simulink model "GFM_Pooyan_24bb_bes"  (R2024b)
settings: Solver=FixedStepAuto  StartTime=0.0  StopTime=1  FixedStep=Ts  RelTol=1e-3
model workspace (MAT data in the model file):
  Po = 0
  b1 = 1000.38104695
  b2 = 1006.47399607
  b3 = 1006.95432939
  b4 = 996.322108769
  b5 = 995.669039411
  b6 = 1012.96535236
  b7 = 1007.5422409
  b8 = 993.960341463
  l1 = 8282.83466164
  l10 = 5511.54621883
  l11 = 8516.9845943
  l12 = 3533.51403234
  l13 = 1255.67117866
  l14 = 1105.23671469
  l15 = 955.492069576
  l16 = 1255.83166019
  l2 = 7767.51754481
  l3 = 6680.69860842
  l4 = 3013.93364227
  l5 = 912.604633733
  l6 = 706.803488619
  l7 = 1117.39027011
  l8 = 1674.30810947
  l9 = 1971.00014576
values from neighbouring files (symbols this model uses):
  alpha_p = 0.0005    [initialcondition_gfm_Pooyan.m]    (also in initialcondition_Pooyan.m = 0.0001)
  alpha_q = 0.0001    [initialcondition_gfm_Pooyan.m]    (also in initialcondition_Pooyan.m)
  Cf = 50e-6    (= 5e-05)    [initialcondition_gfm_Pooyan.m]    (also in initialcondition_Pooyan.m)
  I_instant_limit_peak = I_instant_limit_rms * sqrt(2)    [initialcondition_gfm_Pooyan.m]
  I_overload_limit = 1.2 * I_rated_rms    [initialcondition_gfm_Pooyan.m]
  Kicc = 314.159    [initialcondition_gfm_Pooyan.m]    (also in initialcondition_Pooyan.m)
  Kivc = 400    [initialcondition_gfm_Pooyan.m]    (also in initialcondition_Pooyan.m)
  Kpcc = 31.4159    [initialcondition_gfm_Pooyan.m]    (also in initialcondition_Pooyan.m)
  Kpvc = 0.5    [initialcondition_gfm_Pooyan.m]    (also in initialcondition_Pooyan.m)
  Lf = 10e-3    (= 0.01)    [initialcondition_gfm_Pooyan.m]    (also in initialcondition_Pooyan.m)
  Lg = X_BY_R*Rg/(wn)    [initialcondition_gfm_Pooyan.m]    (also in DER_param.m = (X_BY_R_gfl * Rg) / wn_gfl; initialcondition_Pooyan.m)
  Pn = 20000    [initialcondition_gfm_Pooyan.m]    (also in initialcondition_Pooyan.m)
  Qn = 0    [initialcondition_gfm_Pooyan.m]    (also in initialcondition_Pooyan.m)
  R = (3*Vg^2)/(2*Pn)    (= 8.000067)    [initialcondition_gfm_Pooyan.m]    (also in MC2.m = (8760*SS-sum(Tdown))/(8760*SS); initialcondition_Pooyan.m)
  R_extra = (3*Vg^2)/(2*P_extra)    (= 10.666756)    [initialcondition_gfm_Pooyan.m]
  Rf = 0.1    [initialcondition_gfm_Pooyan.m]    (also in initialcondition_Pooyan.m)
  Rg = (3*Vg^2)/(2*SCR*sqrt(1+X_BY_R^2)*Pn)    [initialcondition_gfm_Pooyan.m]    (also in DER_param.m = (3 * Vg_gfl^2) / (2 * SCR_gfl * sqrt(1 + X_BY_R_gfl^2) * Pn_; initialcondition_Pooyan.m)
  tau_p = 0.031415    [initialcondition_gfm_Pooyan.m]    (also in initialcondition_Pooyan.m)
  tau_q = 0.031415    [initialcondition_gfm_Pooyan.m]    (also in initialcondition_Pooyan.m)
  Ts = 50e-6    (= 5e-05)    [initialcondition_gfm_Pooyan.m]    (also in initialcondition_Pooyan.m)
  Vdc = 700    [initialcondition_gfm_Pooyan.m]    (also in initialcondition_Pooyan.m)
  Vg = 326.6    [initialcondition_gfm_Pooyan.m]    (also in initialcondition_Pooyan.m)
  wn = 2*pi*50    (= 314.159265359)    [initialcondition_gfm_Pooyan.m]    (also in initialcondition_Pooyan.m)
undefined symbols (not defined in the file or in its folder): Ion, Lithium
libraries: simulink x6, slpidlib x5, spsThreePhaseBreakerLib x3, spsabctodq0Lib x3, spsGroundLib x3, spsThreePhaseSeriesRLCBranchLib x3, spsThreePhaseVIMeasurementLib x3, spsIGBTDiodeLib x2, spsSeriesRLCBranchLib x2, spsThreePhaseParallelRLCBranchLib x2, spsThreePhaseSourceLib x1, spsBatteryLib x1
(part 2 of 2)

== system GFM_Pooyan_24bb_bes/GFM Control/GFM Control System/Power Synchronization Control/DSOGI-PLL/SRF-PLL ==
  al-be-0 : Inport
  1/2/pi : Gain  Gain=1/(2*pi)
  2 : Constant  Value=2*pi
  3 : Constant  Value=0
  Al_Be_0 to dq0 : Subsystem
  Integrator : Integrator
  Math Function : Math  Operator=mod  SignedPower=on
  "PI " : slpidlib/PID Controller  Controller=PI  Form=Parallel  TimeDomain=Continuous-time  UseExternalTs=off  SampleTime=100e-6  IntegratorMethod=Forward Euler  FilterMethod=Forward Euler  ControllerParametersSource=internal  P=10  I=30  UseKiTs=off  D=0  UseExternalDerivativeSource=off  N=100  UseFilter=on  TunerSelectOption=Transfer Function Based (PID Tuner App)  InitialConditionSource=internal  InitialConditionForIntegrator=0  InitialConditionForFilter=0  DifferentiatorICPrevScaledInput=0  ExternalReset=none  TrackingMode=off  Kt=1  LimitOutput=off  SatLimitsSource=internal  UpperSaturationLimit=inf  LowerSaturationLimit=-inf  LinearizeAsGain=on  AntiWindupMode=none  Kb=1  LimitIntegrator=off  UpperIntegratorSaturationLimit=inf  LowerIntegratorSaturationLimit=-inf  POutMin=[]  POutMax=[]  IOutMin=[]  IOutMax=[]  DOutMin=[]  DOutMax=[]  NOutMin=[]  NOutMax=[]  SumOutMin=[]  SumOutMax=[]  SaturationOutMin=[]  SaturationOutMax=[]  PParamMin=[]  PParamMax=[]  IParamMin=[]  IParamMax=[]  DParamMin=[]  DParamMax=[]  NParamMin=[]  NParamMax=[]  KbParamMin=[]  KbParamMax=[]  KtParamMin=[]  KtParamMax=[]  KbOutMin=[]  KbOutMax=[]  KtOutMin=[]  KtOutMax=[]  IntegratorOutMin=[]  IntegratorOutMax=[]  FilterOutMin=[]  FilterOutMax=[]  SumI1OutMin=[]  SumI1OutMax=[]  SumI2OutMin=[]  SumI2OutMax=[]  SumI3OutMin=[]  SumI3OutMax=[]  SumI4OutMin=[]  SumI4OutMax=[]  SumDOutMin=[]  SumDOutMax=[]  DifferentiatorOutMin=[]  DifferentiatorOutMax=[]  FilterDiffOutCoefMin=[]  FilterDiffOutCoefMax=[]  ReciprocalOutMin=[]  ReciprocalOutMax=[]  SumDenOutMin=[]  SumDenOutMax=[]  SumNumOutMin=[]  SumNumOutMax=[]  DivideOutMin=[]  DivideOutMax=[]  UdiffTsProdOutMin=[]  UdiffTsProdOutMax=[]  NTsProdOutMin=[]  NTsProdOutMax=[]  UintegralTsProdOutMin=[]  UintegralTsProdOutMax=[]  UngainTsProdOutMin=[]  UngainTsProdOutMax=[]  ClampingZeroOutDataTypeStr=Inherit: Inherit via back propagation  ClampingZeroOutMin=[]  ClampingZeroOutMax=[]  FilterDenConstantOutDataTypeStr=Inherit: Inherit via back propagation  FilterDenConstantOutMin=[]  FilterDenConstantOutMax=[]  PCopyOutDataTypeStr=Inherit: Inherit via back propagation  PCopyOutMin=[]  PCopyOutMax=[]  NCopyOutDataTypeStr=Inherit: Inherit via back propagation  NCopyOutMin=[]  NCopyOutMax=[]  IntegratorContinuousStateAttributes=''  IntegratorStateMustResolveToSignalObject=off  IntegratorRTWStateStorageClass=Auto  FilterContinuousStateAttributes=''  FilterStateMustResolveToSignalObject=off  FilterRTWStateStorageClass=Auto  ParallelPVariant=InternalParameters  IdealPVariant=Disabled  IVariant=InternalParameters  DVariant=Disabled  IntegratorVariant=Continuous  SatVariant=Disabled  AWVariant=Passthrough  PCopyVariant=Disabled  TRVariant=Disabled  FdbkBlocksVariant=Forward  IdealPFdbkVariant=Disabled  SatFdbkVariant=Disabled  DerivativeFilterVariant=Disabled  NVariant=Disabled  NCopyVariant=Disabled_SignalSpec  FilterICVariant=Disabled  IntegratorICVariant=InternalICs  ExternalResetVariant=Disabled  TRSumVariant=Passthrough  SumFdbkVariant=Disabled  SumVariant=Sum_PI  TsampFilterVariant=InternalTs  TsampNgainVariant=Passthrough  TsampIntegralVariant=Disabled_SignalSpec  ExternalSaturationOutDataTypeStr=Inherit: Same as second input  DerivativeSourceVariant=Disabled  PreIntVariant=InternalPreInt
  Second-Order Filter : spsSecondOrderFilterLib/Second-Order Filter  FilterType=Lowpass  Fo=5  Zeta=0.707  Ts=0  Initialize=off  Vac_Init="[0,  0,  50]"  Vdc_Init=0  PlotResponse=off  FreqRange=[0, 500, 1]
  Selector : Selector  InputPortWidth=3  IndexOptions=Index vector (dialog)  Indices=1  OutputSizes=1
  Sum1 : Sum  Inputs=|++
  Sum2 : Sum  Inputs=|+-
  w : Constant  Value=100*pi
  theta_pcc : Outport  VectorParamsAs1DForOutWhenUnconnected=off
  f : Outport  Port=2  VectorParamsAs1DForOutWhenUnconnected=off
  w_pcc : Outport  Port=3  VectorParamsAs1DForOutWhenUnconnected=off
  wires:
  1/2/pi/1 -> Second-Order Filter/1
  Integrator/1 -> Al_Be_0 to dq0/2(wt), theta_pcc/1, Math Function/1
  2/1 -> Math Function/2
  Sum1/1 -> Integrator/1, w_pcc/1, 1/2/pi/1
  w/1 -> Sum1/2
  "PI "/1 -> Sum1/1
  Sum2/1 -> "PI "/1
  al-be-0/1 -> Al_Be_0 to dq0/1(Al_Be_0)
  3/1 -> Sum2/2
  Al_Be_0 to dq0/1(dq0) -> Selector/1
  Selector/1 -> Sum2/1
  Second-Order Filter/1 -> f/1

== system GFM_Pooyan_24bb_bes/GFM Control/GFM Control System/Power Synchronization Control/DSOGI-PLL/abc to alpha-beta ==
  abc : Inport
  Gain1 : Gain  Gain=(2/3)  SaturateOnIntegerOverflow=on
  Gain3 : Gain  Gain="[ 1   -1/2   -1/2; 0   sqrt(3)/2   -sqrt(3)/2 ]"  Multiplication=Matrix(K*u) (u vector)  SaturateOnIntegerOverflow=on
  al_be : Outport  VectorParamsAs1DForOutWhenUnconnected=off
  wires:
  abc/1 -> Gain3/1
  Gain1/1 -> al_be/1
  Gain3/1 -> Gain1/1

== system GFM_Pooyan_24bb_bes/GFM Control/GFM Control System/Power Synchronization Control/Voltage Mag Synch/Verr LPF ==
  In : Inport
  Add : Sum  Inputs=+-
  Constant1 : Constant  Value=1 / (2*pi*fc)
  Constant2 : Constant
  Constant3 : Constant
  Divide : Product  Inputs=*/
  LPF : Subsystem  mask(Basic IIR LPF filter){}
      mask help: The output is computed as: y[k] = G * y[k-1] + (1-G) * u[k]
  Weighted Sample Time1 : SampleTimeMath
  Weighted Sample Time2 : SampleTimeMath  TsampMathOp=Ts Only
  Out : Outport
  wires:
  Constant3/1 -> Weighted Sample Time2/1
  Divide/1 -> Add/2  "α"
  Weighted Sample Time2/1 -> Divide/1
  Weighted Sample Time1/1 -> Divide/2
  Constant1/1 -> Weighted Sample Time1/1
  Constant2/1 -> Add/1
  In/1 -> LPF/1(In)
  LPF/1(Out) -> Out/1
  Add/1 -> LPF/2(G)

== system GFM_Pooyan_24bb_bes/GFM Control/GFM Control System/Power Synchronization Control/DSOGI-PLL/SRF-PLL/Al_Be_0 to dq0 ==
  Al_Be_0 : Inport
  wt : Inport  Port=2
  Fcn : Fcn  Expr=u[1]*cos(u[4]) + u[2]*sin(u[4])
  Fcn1 : Fcn  Expr=-u[1]*sin(u[4]) + u[2]*cos(u[4])
  Fcn2 : Fcn  Expr=u[3]
  Mux1 : Mux  Inputs=[3 1]
  Mux2 : Mux  Inputs=3
  dq0 : Outport  VectorParamsAs1DForOutWhenUnconnected=off
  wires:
  Mux1/1 -> Fcn/1, Fcn2/1, Fcn1/1
  Fcn1/1 -> Mux2/2
  wt/1 -> Mux1/2
  Mux2/1 -> dq0/1
  Al_Be_0/1 -> Mux1/1
  Fcn2/1 -> Mux2/3
  Fcn/1 -> Mux2/1

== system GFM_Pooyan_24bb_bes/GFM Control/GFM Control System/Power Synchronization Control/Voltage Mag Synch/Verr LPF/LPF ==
  In : Inport
  G : Inport  Port=2
  Add : Sum  Inputs=|++
  Constant : Constant  OutDataTypeStr=Inherit: Inherit via back propagation
  Data Type Conversion : DataTypeConversion  OutDataTypeStr=single
  Delay : Delay  DelayLength=1
  Minus : Sum  Inputs=+-
  Product : Product
  Product1 : Product
  Out : Outport
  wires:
  Minus/1 -> Product/2
  G/1 -> Minus/2, Product1/1
  Constant/1 -> Minus/1
  Delay/1 -> Product1/2
  In/1 -> Product/1
  Product/1 -> Add/1
  Product1/1 -> Add/2
  Add/1 -> Data Type Conversion/1, Delay/1
  Data Type Conversion/1 -> Out/1

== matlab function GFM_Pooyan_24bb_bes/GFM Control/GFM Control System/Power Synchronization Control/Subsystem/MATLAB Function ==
function y = fcn(error,error_w,reset)
out=single(error);
e_w=single(error_w);
band=single(0.2*2*pi);  % Threshold is 0.2Hz or 1.2566

if reset==0 && abs(e_w)<=band 
	out=single(error);
else
    out=single(0);
end
y = single(out);

end

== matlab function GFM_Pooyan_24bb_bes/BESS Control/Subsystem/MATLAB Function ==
function [control_signal,MAX_CURRENT] = fcn(error, Kp, Ki, dt)

% Define a persistent variable to store the integrator state
persistent integrator_state;

% Initialize the persistent variable on the first run
if isempty(integrator_state)
    integrator_state = 0.0;
end

% --- Define Saturation Limits ---
i_fac=1.2;
MAX_CURRENT = 52.0*i_fac;
MIN_CURRENT = -MAX_CURRENT ; % Or a negative value if charging is allowed

% --- PI Controller Calculation ---
p_term = Kp * error;
unsaturated_output = p_term + integrator_state;

% --- Apply Saturation and Anti-Windup ---
[control_signal, new_i_state] = apply_anti_windup(unsaturated_output, error, integrator_state, Ki, dt, MAX_CURRENT, MIN_CURRENT);

% --- Update the state for the next time step ---
integrator_state = new_i_state;

end


% helper function
function [final_output, new_integrator_state] = apply_anti_windup(unsaturated_output, error, integrator_state, Ki, dt, max_limit, min_limit)
    if unsaturated_output > max_limit
        final_output = max_limit;
    elseif unsaturated_output < min_limit
        final_output = min_limit;
    else
        final_output = unsaturated_output;
    end
    
    allow_integration = true;
    if (final_output >= max_limit) && (error > 0)
        allow_integration = false;
    end
    if (final_output <= min_limit) && (error < 0)
        allow_integration = false;
    end
    
    if allow_integration
        new_integrator_state = integrator_state + Ki * error * dt;
    else
        new_integrator_state = integrator_state;
    end
end

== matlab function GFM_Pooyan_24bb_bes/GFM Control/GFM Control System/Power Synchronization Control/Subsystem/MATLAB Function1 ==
function y = fcn(u, sync)
% u: Input from the PI controller
% sync: Synchronization ON (1) or OFF (0) signal

% 1. Declare a persistent variable to store the last output when sync was ON.
persistent last_u_value;

% Initialize the persistent variable on the first call
if isempty(last_u_value)
    last_u_value = single(0);
end

on = single(sync);

if on == 1
    % 2. Mode: Pre-synchronization ON (Relay is Open)
    % The output tracks the PI controller output (u) and saves it.
    out = single(u);
    last_u_value = out; % Continuously update the value to be held
else
    % 3. Mode: Pre-synchronization OFF (Relay is Closed)
    % The output is the last value saved when sync was ON.
    % The PI controller's input should already be zero as per your design.
    out = last_u_value; 
end

y = out;

end

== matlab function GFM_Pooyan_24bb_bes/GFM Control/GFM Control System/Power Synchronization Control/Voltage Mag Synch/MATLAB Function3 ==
function y = fcn(u,sync)
on=single(sync);

if on==0
    out=single(0);
else
    out=single(u);
end

y = out;


% function y = fcn(u, sync)
% % u: Input from the PI controller
% % sync: Synchronization ON (1) or OFF (0) signal
% 
% % 1. Declare a persistent variable to store the last output when sync was ON.
% persistent last_u_value;
% 
% % Initialize the persistent variable on the first call
% if isempty(last_u_value)
%     last_u_value = single(0);
% end
% 
% on = single(sync);
% 
% if on == 1
%     % 2. Mode: Pre-synchronization ON (Relay is Open)
%     % The output tracks the PI controller output (u) and saves it.
%     out = single(u);
%     last_u_value = out; % Continuously update the value to be held
% else
%     % 3. Mode: Pre-synchronization OFF (Relay is Closed)
%     % The output is the last value saved when sync was ON.
%     % The PI controller's input should already be zero as per your design.
%     out = last_u_value; 
% end
% 
% y = out;
% 
% end

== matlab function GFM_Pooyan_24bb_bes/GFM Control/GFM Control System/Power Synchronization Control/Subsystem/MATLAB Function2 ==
function y = fcn(u, sync)
% u: Input from the PI controller
% sync: Synchronization ON (1) or OFF (0) signal

% 1. Declare a persistent variable to store the last output when sync was ON.
persistent last_u_value;

% Initialize the persistent variable on the first call
if isempty(last_u_value)
    last_u_value = single(0);
end

on = single(sync);

if on == 1
    % 2. Mode: Pre-synchronization ON (Relay is Open)
    % The output tracks the PI controller output (u) and saves it.
    out = single(u);
    last_u_value = out; % Continuously update the value to be held
else
    % 3. Mode: Pre-synchronization OFF (Relay is Closed)
    % The output is the last value saved when sync was ON.
    % The PI controller's input should already be zero as per your design.
    out = last_u_value; 
end

y = out;

end

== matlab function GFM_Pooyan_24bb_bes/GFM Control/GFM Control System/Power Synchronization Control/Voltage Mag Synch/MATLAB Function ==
function y = fcn(error,reset)
out=single(error);

if reset==0
    out=single(error);
else
    out=single(0);
end

y = single(out);
end

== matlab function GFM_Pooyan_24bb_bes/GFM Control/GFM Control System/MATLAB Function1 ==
function y = dynamic_gain(u, Vdc_filtered) % Note the input name change
%#codegen
Vdc_min = 10; 
gain = 2 / max(Vdc_filtered, Vdc_min); % Use the filtered value
y = gain .* u;
end
